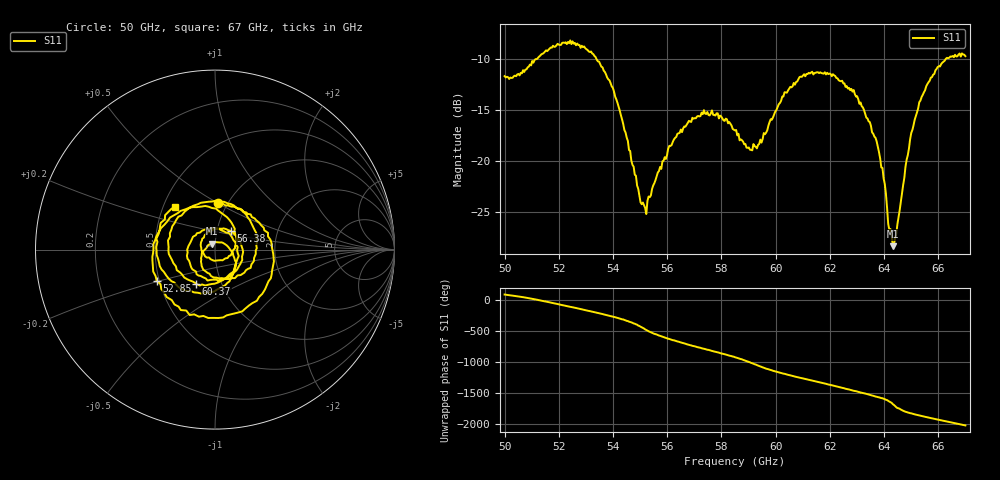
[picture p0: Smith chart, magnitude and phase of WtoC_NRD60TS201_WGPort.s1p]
!Agilent Technologies,E8361A,US42410132,A.06.03.05
!Agilent E8361A: A.06.03.05
!Date: Friday, July 11, 2008 15:48:30
!Correction: S11(Full 2 Port(1,2))
!S1P File: Measurement: S11:
# Hz S  MA  R 50
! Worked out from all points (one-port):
!   401 points, 50 GHz to 67 GHz, reference 50 ohm
!   lowest |S11| = -28.4 dB at 64.32 GHz (marker M1), VSWR 1.08, Z = 48.2 + j3.27 ohm
!   |S11| at or under -10 dB: start of sweep to 51.14 GHz; 53.39 GHz to 66.27 GHz (12.88 GHz wide, 21.5 % of centre)
!   S11 on the Smith chart (normalised r, x): 50 GHz: 0.90, +0.50; 52.85 GHz: 0.48, -0.19; 56.38 GHz: 1.16, +0.25; 60.37 GHz: 0.76, -0.30; 67 GHz: 0.58, +0.31
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5e10  0.2611 86.8
5.0765e10  0.2811 38.1
5.13175e10  0.3297 -8.0
5.2125e10  0.3807 -83.1
5.28475e10  0.3681 -152.0
5.36125e10  0.2887 131.7
5.425e10  0.1765 58.8
5.51425e10  0.06063 -101.8
5.5695e10  0.08921 144.6
5.6375e10  0.136 49.8
5.69275e10  0.163 -21.2
5.7565e10  0.1675 -92.7
5.85e10  0.1413 153.7
5.89675e10  0.116 86.1
5.952e10  0.1281 -8.7
6.037e10  0.2172 -119.0
6.0625e10  0.2327 -146.9
6.1135e10  0.2675 160.2
6.173e10  0.2693 98.2
6.22825e10  0.2548 40.6
6.275e10  0.2227 -12.0
6.32175e10  0.1833 -63.7
6.37275e10  0.1246 -123.6
6.43225e10  0.03811 117.1
6.4875e10  0.1067 -17.8
6.5895e10  0.2789 -124.0
6.64475e10  0.3261 -174.6
6.7e10  0.3273 132.9
